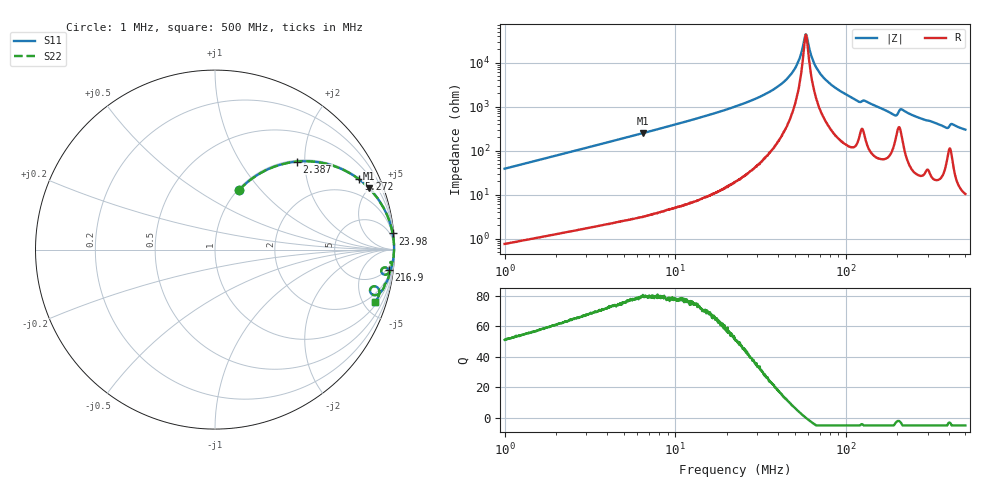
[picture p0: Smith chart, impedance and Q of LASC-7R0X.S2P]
!s-Parameter Generated by FASTRON Sdn. Bhd.
!FASTRON P/N : LASC-7R0X
!Keysight Technologies,E4991B,MY54100416,A.01.15
!Date: Tue Mar 17 10:03:05 2026
!Version  : Rev00 Tue Mar 17 10:03:05 2026
!Data & Calibration Information:
!PortZ  Port1:50+j0  Port2:50+j0
!When reading, reference impedance value at option line is always used.
! Remarks : This data is being provided solely for informational purposes.
!Freq	S11	S21	S12	S22
# Hz S dB R 50
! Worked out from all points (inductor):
!   1601 points, 1 MHz to 500 MHz, reference 50 ohm
!   read as one part in series: L = 6.14 uH near 1.032 MHz
!   highest Q = 79.7 at 6.452 MHz (marker M1), where L = 6.14 uH
!   self-resonance near 58.14 MHz
!   S11 on the Smith chart (normalised r, x): 1 MHz: 1.02, +0.77; 2.387 MHz: 1.03, +1.84; 5.272 MHz: 1.05, +4.06; 23.98 MHz: 1, +22; 216.9 MHz: 4, -16; 500 MHz: 1.21, -5.98
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1000000  -8.90 67.8  -0.66 -21.0  -0.66 -21.0  -8.90 67.8
2387019  -3.47 47.0  -2.72 -42.1  -2.72 -42.1  -3.47 47.0
2820919  -2.74 42.3  -3.44 -46.8  -3.44 -46.8  -2.74 42.3
5271989  -0.99 26.1  -7.13 -63.2  -7.13 -63.2  -0.99 26.1
6451950  -0.69 21.8  -8.61 -67.5  -8.61 -67.5  -0.69 21.8
7957584  -0.47 17.9  -10.26 -71.4  -10.26 -71.4  -0.47 17.9
2.236068e7  -0.06 5.7  -20.02 -83.2  -20.02 -83.2  -0.06 5.7
2.397996e7  -0.05 5.2  -20.85 -83.6  -20.85 -83.6  -0.05 5.2
3.522469e7  -0.03 2.7  -26.49 -85.0  -26.49 -85.0  -0.03 2.7
4.499032e7  -0.02 1.3  -32.54 -83.8  -32.54 -83.8  -0.02 1.3
5.174233e7  -0.02 0.6  -39.25 -78.2  -39.25 -78.2  -0.02 0.6
5.79115e7  -0.02 0.0  -52.73 -10.8  -52.73 -10.8  -0.02 0.0
5.950765e7  -0.02 -0.1  -50.23 40.3  -50.23 40.3  -0.02 -0.1
6.307767e7  -0.02 -0.4  -42.28 71.6  -42.28 71.6  -0.02 -0.4
7.087308e7  -0.02 -1.0  -34.78 80.6  -34.78 80.6  -0.02 -1.0
8.573088e7  -0.03 -2.1  -28.77 83.1  -28.77 83.1  -0.03 -2.1
1.16973e8  -0.10 -4.2  -22.59 79.1  -22.59 79.1  -0.10 -4.2
1.77937e8  -0.18 -7.4  -17.73 77.0  -17.73 77.0  -0.18 -7.4
2.169182e8  -0.22 -6.7  -18.49 74.3  -18.49 74.3  -0.22 -6.7
3.780214e8  -0.59 -15.7  -11.31 68.4  -11.31 68.4  -0.59 -15.7
4.181909e8  -0.59 -13.3  -12.63 67.2  -12.63 67.2  -0.59 -13.3
5e8  -0.55 -18.3  -10.06 69.7  -10.06 69.7  -0.55 -18.3
